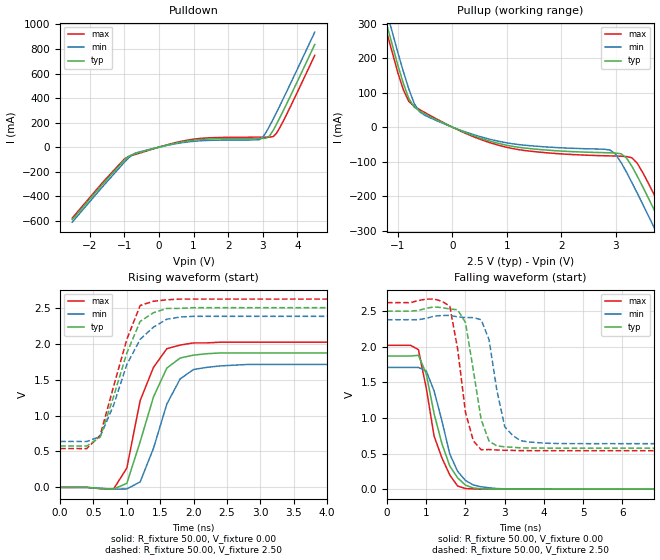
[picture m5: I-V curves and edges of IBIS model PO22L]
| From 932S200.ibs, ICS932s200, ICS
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|   Model PO22L
[Model]   PO22L
Model_type   Output
Polarity   Non-Inverting
Vmeas =   1.50V
Cref =  20.00pF
Rref =  0.000
Vref =   1.50V
C_comp   5.50pF   5.00pF   6.00pF
[Temperature Range]   27.00   70.00   0.00
[Voltage Range]   2.50V   2.38V   2.62V
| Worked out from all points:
|   slope of the pulldown table from 0 to 0.375 V, typ, clamps not added: 14.2 ohm
|   slope of the pullup table from 0 to 0.375 V, typ, clamps not added: 15.6 ohm
|   rising waveform, R_fixture 50.00, V_fixture 0.00: 20-80 % time 408ps typ, 406ps min, 348ps max; typ from 0 V to 1.87 V
|   rising waveform, R_fixture 50.00, V_fixture 2.50: 20-80 % time 418ps typ, 455ps min, 392ps max; typ from 0.576 V to 2.5 V
|   falling waveform, R_fixture 50.00, V_fixture 0.00: 20-80 % time 524ps typ, 519ps min, 501ps max; typ from 1.87 V to 0 V
|   falling waveform, R_fixture 50.00, V_fixture 2.50: 20-80 % time 343ps typ, 338ps min, 340ps max; typ from 2.5 V to 0.576 V
[Pulldown]
| voltage   I(typ)   I(min)   I(max)
-2.5V     -590.6mA   -611.4mA   -577.7mA
-1V       -105.9mA   -124.1mA   -97.14mA
-700mV    -54.98mA   -50.77mA   -60.73mA
200mV     14.72mA    12.47mA    16.51mA
1V        57.25mA    47.93mA    65.12mA
2.8V      70.98mA    59.29mA    81.4mA
3V        71.45mA    81.67mA    81.85mA
3.2V      93.46mA    174.6mA    82.4mA
3.3V      137.1mA    229mA      86.26mA
3.4V      189.4mA    285.4mA    115.2mA
3.7V      359.9mA    459.7mA    274.2mA
4.5V      837.2mA    938.1mA    749.1mA
[Pullup]
| voltage   I(typ)   I(min)   I(max)
-2.5V     1.06A      1.1A       1.04A
-1.6V     525mA      563mA      501.4mA
-1V       178.9mA    215.4mA    157mA
-700mV    57.8mA     68.35mA    60.35mA
300mV     -19.72mA   -17.12mA   -21.96mA
1.3V      -60.1mA    -51.95mA   -67.19mA
2.9V      -74.43mA   -66.47mA   -83.39mA
3.3V      -113.9mA   -161.1mA   -88.89mA
3.7V      -237.5mA   -289mA     -193.5mA
3.9V      -302.8mA   -354.6mA   -258mA
4V        -335.7mA   -387.7mA   -290.8mA
4.5V      -502.1mA   -554.1mA   -456.8mA
[Ramp]
| variable   typ   min   max
dV/dt_r   1.12/296.18p   1.02/367.13p   1.21/273.42p
dV/dt_f   1.15/300.00p   1.05/400.00p   1.25/200.00p
[Rising Waveform]
R_fixture = 50.00
V_fixture = 0.00
V_fixture_min = 0.00
V_fixture_max = 0.00
| time   V(typ)   V(min)   V(max)
0s        0V         0V         0V
800ps     -23.72mV   -24.44mV   -23.5mV
1ns       56.74mV    -21.33mV   269mV
1.2ns     635.6mV    76.76mV    1.21V
1.4ns     1.26V      545.2mV    1.67V
1.6ns     1.66V      1.16V      1.93V
1.8ns     1.8V       1.51V      1.98V
2ns       1.84V      1.64V      2.01V
2.8ns     1.87V      1.71V      2.02V
10ns      1.87V      1.71V      2.02V
[Rising Waveform]
R_fixture = 50.00
V_fixture = 2.50
V_fixture_min = 2.38
V_fixture_max = 2.62
| time   V(typ)   V(min)   V(max)
0s        576.1mV    639.1mV    540.7mV
400ps     575.6mV    638.5mV    540.3mV
600ps     699mV      707.6mV    723.2mV
800ps     1.26V      1.14V      1.4V
1ns       1.87V      1.71V      2.06V
1.2ns     2.31V      2.06V      2.53V
1.4ns     2.43V      2.23V      2.59V
1.6ns     2.49V      2.34V      2.61V
2ns       2.5V       2.38V      2.62V
10ns      2.5V       2.38V      2.62V
[Falling Waveform]
R_fixture = 50.00
V_fixture = 0.00
V_fixture_min = 0.00
V_fixture_max = 0.00
| time   V(typ)   V(min)   V(max)
0s        1.87V      1.71V      2.02V
800ps     1.88V      1.71V      1.96V
1ns       1.62V      1.66V      1.42V
1.2ns     1.06V      1.38V      745.8mV
1.4ns     638.1mV    957.8mV    438.6mV
1.6ns     325mV      492.9mV    198.3mV
1.8ns     158.8mV    250mV      44.47mV
2.2ns     16.37mV    58.82mV    3.4mV
2.8ns     1.45mV     8.59mV     267uV
10ns      0V         4.03uV     1.02uV
[Falling Waveform]
R_fixture = 50.00
V_fixture = 2.50
V_fixture_min = 2.38
V_fixture_max = 2.62
| time   V(typ)   V(min)   V(max)
0s        2.5V       2.38V      2.62V
1.6ns     2.53V      2.44V      2.57V
1.8ns     2.52V      2.42V      1.97V
2ns       2.34V      2.41V      1.08V
2.2ns     1.67V      2.41V      679mV
2.4ns     976.8mV    2.38V      553.4mV
2.6ns     675.4mV    2.1V       556.8mV
3ns       594.5mV    877.1mV    545.6mV
3.4ns     580.5mV    681.7mV    541.9mV
10ns      576.1mV    639.1mV    540.7mV
